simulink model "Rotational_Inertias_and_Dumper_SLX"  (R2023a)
settings: Solver=ode23s  StartTime=0.0  StopTime=10.0  MaxStep=0.001  RelTol=1e-3
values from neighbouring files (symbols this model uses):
  b_3 = 0.1*Nm/(rad/sec)    (= 0.1)    [Rotational_Inertias_and_Dumper_EQN.m]    (also in Rotational_Inertias_and_Dumper_SLX_m.m; Car_Dumper_EQN.m = 2; Car_Dumper_SLX_m.m = 2; Mechanical_Mass_Spring_Mass_EQN.m = 2)
  b_6 = 0.1*Nm/(rad/sec)    (= 0.1)    [Rotational_Inertias_and_Dumper_EQN.m]    (also in Rotational_Inertias_and_Dumper_SLX_m.m; Car_Dumper_EQN.m = 2; Car_Dumper_SLX_m.m = 2; Mechanical_Mass_Spring_Mass_EQN.m = 2)
  b_7 = 0.1*Nm/(rad/sec)    (= 0.1)    [Rotational_Inertias_and_Dumper_EQN.m]    (also in Rotational_Inertias_and_Dumper_SLX_m.m; Car_Dumper_EQN.m = 2; Car_Dumper_SLX_m.m = 2; Electrical_DC_Motor_EQN.m)
  J_2 = 0.01*kg*m^2    (= 0.01)    [Rotational_Inertias_and_Dumper_EQN.m]    (also in Rotational_Inertias_and_Dumper_SLX_m.m; Mechanical_system_EQN.m; Mechanical_system_SLX_m.m)
  J_5 = 0.01*kg*m^2    (= 0.01)    [Rotational_Inertias_and_Dumper_EQN.m]    (also in Rotational_Inertias_and_Dumper_SLX_m.m)
  K_4 = 10*Nm/rad    (= 10)    [Rotational_Inertias_and_Dumper_EQN.m]    (also in Rotational_Inertias_and_Dumper_SLX_m.m; Car_Dumper_EQN.m = 1000; Car_Dumper_SLX_m.m = 1000; Mechanical_Mass_Spring_Mass_EQN.m = 1000)
  K_8 = 10*Nm/rad    (= 10)    [Rotational_Inertias_and_Dumper_EQN.m]    (also in Rotational_Inertias_and_Dumper_SLX_m.m; Car_Dumper_EQN.m = 1000; Car_Dumper_SLX_m.m = 1000; Hydraulic_Clutch_System_EQN.m = 1000)
  T_1_0 = 10*Nm    (= 10)    [Rotational_Inertias_and_Dumper_SLX_m.m]    (also in Mechanical_system_SLX_m.m)
  T_4_0 = 0*Nm    (= 0)    [Rotational_Inertias_and_Dumper_SLX_m.m]
  T_8_0 = 0*Nm    (= 0)    [Rotational_Inertias_and_Dumper_SLX_m.m]    (also in Electrical_DC_Motor_SLX_m.m)
  Ts = Tfin/Nr_Ts_Points    (= 0.00090885)    [Rotational_Inertias_and_Dumper_SLX_m.m]    (also in BIG_EC_Simscape_SLX_m.m = 0.0003; Car_Dumper_SLX_m.m = 0.0022779; Electric_Circuit_01_SLX_m.m = 0.005; Electric_Circuit_02_SLX_m.m = 0.000480145)
  w_2_0 = 0*rad/sec    (= 0)    [Rotational_Inertias_and_Dumper_SLX_m.m]    (also in Mechanical_system_SLX_m.m)
  w_5_0 = 0*rad/sec    (= 0)    [Rotational_Inertias_and_Dumper_SLX_m.m]
  w_9_0 = 0*rad/sec    (= 0)    [Rotational_Inertias_and_Dumper_SLX_m.m]

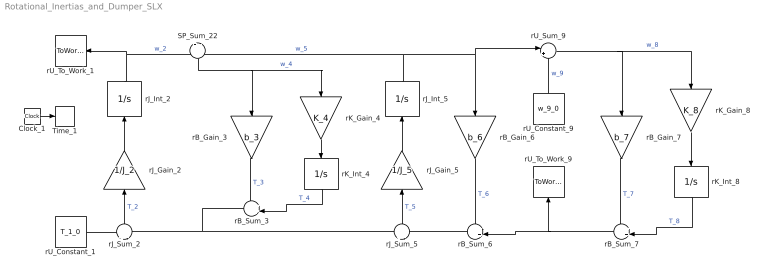
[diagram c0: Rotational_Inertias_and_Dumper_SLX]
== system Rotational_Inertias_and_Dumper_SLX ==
  Clock_1 : Clock
  SP_Sum_22 : Sum  Inputs=+|-
  Time_1 : ToWorkspace  VariableName=t  SaveFormat=Timeseries  SampleTime=Ts
  rB_Gain_3 : Gain  Gain=b_3  Multiplication=Matrix(K*u)
  rB_Gain_6 : Gain  Gain=b_6  Multiplication=Matrix(K*u)
  rB_Gain_7 : Gain  Gain=b_7  Multiplication=Matrix(K*u)
  rB_Sum_3 : Sum  Inputs=++|
  rB_Sum_6 : Sum  Inputs=++|
  rB_Sum_7 : Sum  Inputs=++|
  rJ_Gain_2 : Gain  Gain=1/J_2  Multiplication=Matrix(K*u)
  rJ_Gain_5 : Gain  Gain=1/J_5  Multiplication=Matrix(K*u)
  rJ_Int_2 : Integrator  InitialCondition=w_2_0
  rJ_Int_5 : Integrator  InitialCondition=w_5_0
  rJ_Sum_2 : Sum  Inputs=+|-
  rJ_Sum_5 : Sum  Inputs=+|-
  rK_Gain_4 : Gain  Gain=K_4  Multiplication=Matrix(K*u)
  rK_Gain_8 : Gain  Gain=K_8  Multiplication=Matrix(K*u)
  rK_Int_4 : Integrator  InitialCondition=T_4_0
  rK_Int_8 : Integrator  InitialCondition=T_8_0
  rU_Constant_1 : Constant  Value=T_1_0
  rU_Constant_9 : Constant  Value=w_9_0
  rU_Sum_9 : Sum  Inputs=|+-
  rU_To_Work_1 : ToWorkspace  VariableName=w_1_0  SaveFormat=Timeseries  SampleTime=Ts
  rU_To_Work_9 : ToWorkspace  VariableName=T_9_0  SaveFormat=Timeseries  SampleTime=Ts
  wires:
  rU_Constant_1/1 -> rJ_Sum_2/1
  rB_Sum_3/1 -> rJ_Sum_2/2, rJ_Sum_5/1
  rJ_Int_2/1 -> rU_To_Work_1/1, SP_Sum_22/1  "w_2"
  rJ_Sum_2/1 -> rJ_Gain_2/1  "T_2"
  rJ_Gain_2/1 -> rJ_Int_2/1
  rJ_Int_5/1 -> SP_Sum_22/2, rB_Gain_6/1, rU_Sum_9/1  "w_5"
  SP_Sum_22/1 -> rB_Gain_3/1, rK_Gain_4/1  "w_4"
  rK_Int_4/1 -> rB_Sum_3/2  "T_4"
  rB_Gain_3/1 -> rB_Sum_3/1  "T_3"
  rK_Gain_4/1 -> rK_Int_4/1
  rB_Sum_6/1 -> rJ_Sum_5/2
  rJ_Sum_5/1 -> rJ_Gain_5/1  "T_5"
  rJ_Gain_5/1 -> rJ_Int_5/1
  rB_Sum_7/1 -> rB_Sum_6/2, rU_To_Work_9/1
  rB_Gain_6/1 -> rB_Sum_6/1  "T_6"
  rU_Sum_9/1 -> rB_Gain_7/1, rK_Gain_8/1  "w_8"
  rU_Constant_9/1 -> rU_Sum_9/2  "w_9"
  rK_Int_8/1 -> rB_Sum_7/2  "T_8"
  rB_Gain_7/1 -> rB_Sum_7/1  "T_7"
  rK_Gain_8/1 -> rK_Int_8/1
  Clock_1/1 -> Time_1/1
